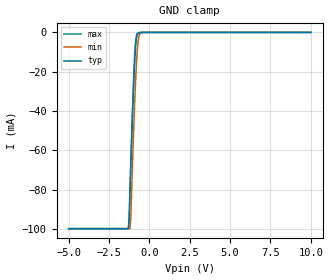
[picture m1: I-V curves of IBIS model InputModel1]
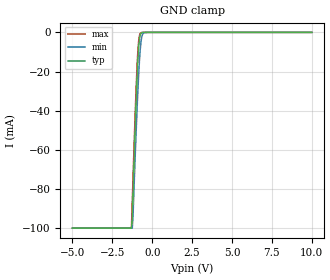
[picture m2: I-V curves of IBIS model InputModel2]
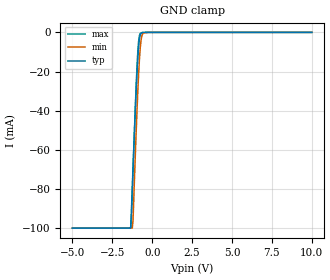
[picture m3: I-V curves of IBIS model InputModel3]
[IBIS Ver]   2.1
[File name]   e_200bv5.ibs   | e_= TSOP, f200bv= abbr chip name, 5= 5V Vcc
[File Rev]   2.00
[Date]   28-February-96
[Source]   File generated from lab measurements at Intel Corporation
[Notes]   Rev 2.00 All data was replaced by actual measurements
   performed in a lab.
[Disclaimer] INTEL DEVELOPER'S SOFTWARE LICENSE AGREEMENT
| BY USING THIS SOFTWARE, YOU ARE AGREEING TO BE BOUND
| BY THE TERMS OF THIS AGREEMENT.  DO NOT USE THE SOFTWARE
| UNTIL YOU HAVE CAREFULLY READ AND AGREED TO THE FOLLOWING
| TERMS AND CONDITIONS.  IF YOU DO NOT AGREE TO THE TERMS
| OF THIS AGREEMENT, PROMPTLY RETURN THE SOFTWARE PACKAGE
| AND ANY ACCOMPANYING ITEMS.
| IF YOU USE THIS SOFTWARE, YOU WILL BE BOUND BY THE TERMS
| OF THIS AGREEMENT
| LICENSE: Intel Corporation ("Intel") grants you the non-exclusive right
| to use the enclosed software program ("Software").  You will not use,
| copy, modify, rent, sell or transfer the Software or any portion
| thereof, except as provided in this Agreement.
| System OEM Developers may:
| 1.   Copy the Software for support, backup or archival purposes;
| 2.   Install, use, or distribute Intel owned Software in object code
|   only;
| 3.   Modify and/or use Software source code that Intel directly makes
|   available to you as an OEM Developer;
| 4.   Install, use, modify, distribute, and/or make or have made
|   derivatives ("Derivatives") of Intel owned Software under the
|   terms and conditions in this Agreement, ONLY if you are a System
|   OEM Developer and NOT an end-user.
| RESTRICTIONS:
| YOU WILL NOT:
| 1.   Copy the Software, in whole or in part, except as provided for
|   in this Agreement;
| 2.   Decompile or reverse engineer any Software provided in object
|   code format;
| 3.   Distribute any Software or Derivative code to any end-users,
|   unless approved by Intel in a prior writing.
| TRANSFER: You may transfer the Software to another OEM
| Developer if the receiving party agrees to the terms of this
| Agreement at the sole risk of any receiving party.
| OWNERSHIP AND COPYRIGHT OF SOFTWARE:
| Title to the Software and all copies thereof remain with Intel
| or its vendors.  The Software is copyrighted and is protected by
| United States and international copyright laws.  You will not
| remove the copyright notice from the Software.  You agree to
| prevent any unauthorized copying of the Software.
| DERIVATIVE WORK: OEM Developers that make or have made
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[Copyright]   Copyright 1996, Intel Corporation, All Rights Reserved
[Component]   E28F200BV   | 56-lead TSOP package, 28F200BV
[Manufacturer]  Intel   | Boot Block (tm)
|   | operating in 5V Vcc range
[Package]
|Variable   typ   min   max
|The following values apply for the Copper leadframe.
R_pkg   48m   41m   54m
L_pkg   4.92nH   4.44nH   5.39nH
C_pkg   0.48pF   0.45pF   0.50pF
|The following values apply for the Alloy-42 leadframe.
|R_pkg   195m   180m   210m
|L_pkg   4.92nH   4.44nH   5.39nH
|C_pkg   0.48pF   0.45pF   0.50pF
|*****************************Pin Definitions*****************************
[Pin]   signal_name   model_name   R_pin   L_pin   C_pin
 1   NC   InputModel4
 2   NC   InputModel4
 3   A15   InputModel3
 4   A14   InputModel3
 5   A13   InputModel3
 6   A12   InputModel3
 7   A11   InputModel3
 8   A10   InputModel3
 9   A09   InputModel1
10   A08   InputModel1
11   NC   InputModel4
12   NC   InputModel4
13   WE#   InputModel1
14   RP#   InputModel1
15   NC   InputModel4
16   NC   InputModel4
17   VPP   POWER
18   WP#   InputModel1
19   NC   InputModel4
20   NC   InputModel3
21   A07   InputModel3
22   A06   InputModel3
23   A05   InputModel3
24   A04   InputModel3
25   A03   InputModel3
26   A02   InputModel3
27   A01   InputModel3
28   NC   InputModel3
29   NC   InputModel4
30   NC   InputModel4
31   A00   InputModel2
32   CE#   InputModel1
33   GND   GND
34   OE#   InputModel1
35   DQ0   InputOutput
36   DQ8   InputOutput
37   DQ1   InputOutput
38   DQ9   InputOutput
39   DQ2   InputOutput
40   DQ10   InputOutput
41   DQ3   InputOutput
42   DQ11   InputOutput
43   VCC   POWER
44   VCC   POWER
45   DQ4   InputOutput
46   DQ12   InputOutput
47   DQ5   InputOutput
48   DQ13   InputOutput
49   DQ6   InputOutput
50   DQ14   InputOutput
51   DQ7   InputOutput
52   DQ15   InputOutput
53   GND   GND
54   BYTE#   InputModel2
55   A16   InputModel2
56   NC   InputModel4
|***********************Input Model 4******************************
[Model]   InputModel4
Model_type   Input
|   Model for all NC pins, excluding NC pin #20.
Vinl = 0.8V
Vinh = 2.0V
|Variable   Typ   Min   Max
C_comp   5.61p   NA   7.6p
[Voltage Range]   5.0V   4.5V   5.5V
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| Models and submodels in the file (5): InputModel1 (Input), InputModel2 (Input), InputModel3 (Input), InputModel4 (Input), InputOutput (I/O)
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|*********************Input Model 1************************************
[Model]   InputModel1
Model_type   Input
|   Model for WE#, WP#, RP#, OE# & CE#.
Vinl = 0.8V
Vinh = 2.0V
|Variable   Typ   Min   Max
C_comp   5.61p   NA   7.6p
[Voltage Range]   5.0V   4.5V   5.5V
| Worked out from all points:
|   GND clamp passes 1 mA (typ) near -0.74 V on its own axis
[GND_clamp]
|Voltage  I(typ)   I(min)   I(max)
-5V       -99.85mA   -99.85mA   -99.85mA
-1.3V     -99.85mA   -99.85mA   -99.85mA
-1.25V    -93.26mA   -99.85mA   -95.79mA
-1.2V     -80.3mA    -99.85mA   -81.5mA
-1.15V    -67.6mA    -94.88mA   -67.39mA
-1V       -32.49mA   -56.57mA   -29.26mA
-900mV    -13.7mA    -33.97mA   -10.19mA
-850mV    -7.324mA   -24.38mA   -4.514mA
-750mV    -1.17mA    -9.368mA   -570.4uA
-650mV    -196.9uA   -2.246mA   -163.7uA
-500mV    -19.68uA   -149.2uA   0A
10V       0A         0A         0A
[Power_clamp]
| Input buffer circuits of this product do not intrinsically
| require a [Power_clamp] definition.  This zero current
| [Power_clamp] table is provided for the compatibility with
| some IBIS parsers.
|Voltage  I(typ)   I(min)   I(max)
-5V       0A         0A         0A
0V        0A         0A         0A
5V        0A         0A         0A
10V       0A         0A         0A
|*********************Input Model 2******************************
[Model]   InputModel2
Model_type   Input
|   Model for A[0], A[16] & BYTE# pins.
Vinl = 0.8V
Vinh = 2.0V
|Variable   Typ   Min   Max
C_comp   5.61p   NA   7.6p
[Voltage Range]   5.0V   4.5V   5.5V
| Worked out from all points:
|   GND clamp passes 1 mA (typ) near -0.74 V on its own axis
[GND_clamp]
|Voltage  I(typ)   I(min)   I(max)
-5V       -99.85mA   -99.85mA   -99.85mA
-1.3V     -99.85mA   -99.85mA   -99.7mA
-1.25V    -95.1mA    -99.85mA   -86.57mA
-1.2V     -81.91mA   -93.12mA   -73.81mA
-1.05V    -44.51mA   -59.81mA   -37.94mA
-950mV    -22.91mA   -39.4mA    -17.7mA
-900mV    -14.12mA   -30.1mA    -9.812mA
-850mV    -7.485mA   -21.87mA   -4.492mA
-750mV    -1.181mA   -8.658mA   -581.8uA
-650mV    0A         -2.149mA   -166uA
-500mV    0A         -145.6uA   -18.8uA
10V       0A         0A         0A
[Power_clamp]
| Input buffer circuits of this product do not intrinsically
| require a [Power_clamp] definition.  This zero current
| [Power_clamp] table is provided for the compatibility with
| some IBIS parsers.
|Voltage  I(typ)   I(min)   I(max)
-5V       0A         0A         0A
0V        0A         0A         0A
5V        0A         0A         0A
10V       0A         0A         0A
|***********************Input Model 3******************************
[Model]   InputModel3
Model_type   Input
|   Model for A[15:1] & NC pin #20.
Vinl = 0.8V
Vinh = 2.0V
|Variable   Typ   Min   Max
C_comp   5.61p   NA   7.6p
[Voltage Range]   5.0V   4.5V   5.5V
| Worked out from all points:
|   GND clamp passes 1 mA (typ) near -0.74 V on its own axis
[GND_clamp]
|Voltage  I(typ)   I(min)   I(max)
-5V       -99.85mA   -99.86mA   -99.85mA
-1.35V    -99.85mA   -99.86mA   -99.85mA
-1.3V     -90.17mA   -99.86mA   -94.83mA
-1.25V    -79.25mA   -99.86mA   -82.83mA
-1.2V     -68.58mA   -95.57mA   -70.38mA
-1.05V    -38.07mA   -60.6mA    -36.34mA
-950mV    -20.19mA   -39.21mA   -17.09mA
-850mV    -7.009mA   -21.02mA   -4.405mA
-750mV    -1.188mA   -7.828mA   -577.2uA
-600mV    -101.4uA   -746.5uA   -94.18uA
-250mV    0A         0A         0A
10V       0A         0A         0A
[Power_clamp]
| Input buffer circuits of this product do not intrinsically
| require a [Power_clamp] definition.  This zero current
| [Power_clamp] table is provided for the compatibility with
| some IBIS parsers.
|Voltage  I(typ)   I(min)   I(max)
-5V       0A         0A         0A
0V        0A         0A         0A
5V        0A         0A         0A
10V       0A         0A         0A
